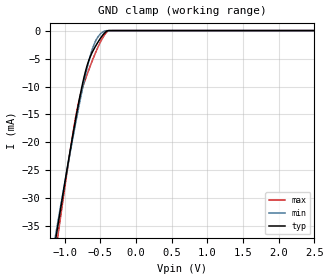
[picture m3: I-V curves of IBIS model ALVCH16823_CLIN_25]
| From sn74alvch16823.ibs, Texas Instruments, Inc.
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[Model]   ALVCH16823_CLIN_25
Model_type  Input
Vinl=0.7
Vinh=1.7
| variable   typ   min   max
C_comp   2.56pF   1.91pF   3.17pF
[Temperature Range]   40   100   -40
| Ambient temperature   25   85   -40
[Voltage range]   2.5   2.3   2.7
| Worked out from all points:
|   GND clamp passes 1 mA (typ) near -0.48 V on its own axis
[GND Clamp]
| ALVCH16823_CLIN_25
|   Voltage   I(typ)   I(min)   I(max)
-2.5V     -153.1mA   -143.6mA   -168.5mA
-1.145V   -38.97mA   -38mA      -41.38mA
-1.11V    -36.17mA   -35.41mA   -38.21mA
-1.08V    -33.78mA   -33.21mA   -35.51mA
-895mV    -19.51mA   -19.99mA   -19.35mA
-800mV    -12.78mA   -13.61mA   -12.64mA
-700mV    -6.981mA   -7.539mA   -8.412mA
-615mV    -3.968mA   -3.483mA   -5.497mA
-540mV    -2.234mA   -1.292mA   -3.196mA
-450mV    -586.7uA   -156.6uA   -959.9uA
-375mV    -85.17nA   -8.524uA   -4.38uA
2.5V      34.28pA    152.6pA    32.5pA
